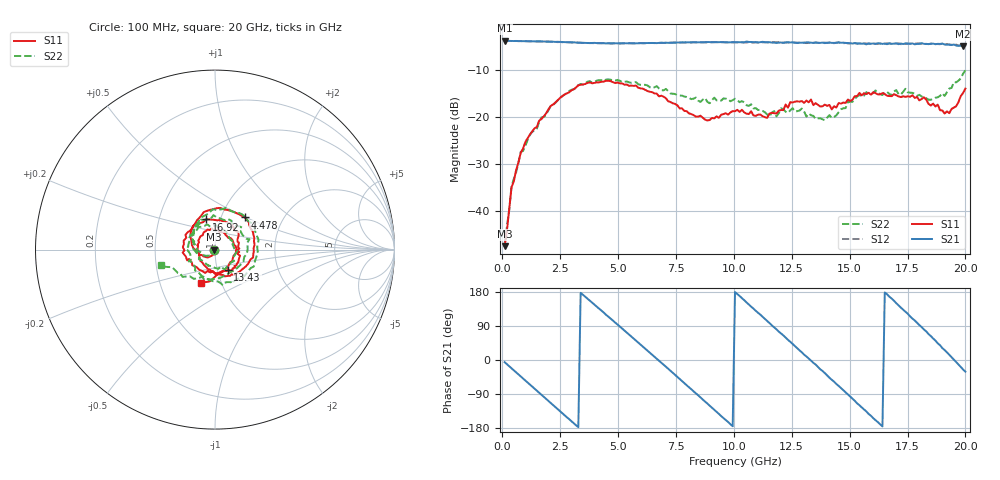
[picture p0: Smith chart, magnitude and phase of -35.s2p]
!Agilent Technologies,N5230C,MY49001569,A.09.33.09
!Agilent N5230C: A.09.33.09
!Date: Wednesday, July 29, 2015 16:57:40
!Correction: S11(Full 2 Port(1,2))
!S21(Full 2 Port(1,2))
!S12(Full 2 Port(1,2))
!S22(Full 2 Port(1,2))
!S2P File: Measurements: S11, S21, S12, S22:
# Hz S  dB  R 50
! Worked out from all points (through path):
!   201 points, 100 MHz to 20 GHz, reference 50 ohm
!   highest |S21| = -3.67 dB at 100 MHz (marker M1); lowest = -4.9 dB at 19.9 GHz (marker M2)
!   group delay of S21, straight-line fit = 153 ps
!   lowest |S11| = -47.6 dB at 100 MHz (marker M3), VSWR 1.01, Z = 49.6 - j0.0396 ohm
!   |S11| at or under -10 dB: start of sweep to end of sweep
!   |S22| runs from -47.3 to -10.0 dB; largest |S21 - S12| = 0.023
!   S11 on the Smith chart (normalised r, x): 100 MHz: 0.99, -0.00; 4.478 GHz: 1.29, +0.49; 13.43 GHz: 1.12, -0.26; 16.92 GHz: 0.86, +0.30; 20 GHz: 0.80, -0.31
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1e8  -47.59 -174.5  -3.67 -5.7  -3.65 -5.9  -47.28 -158.9
3.985e8  -34.99 -91.1  -3.77 -21.9  -3.77 -21.9  -34.74 -91.7
9.955e8  -25.33 -129.2  -3.81 -54.2  -3.80 -54.3  -26.16 -137.0
2.09e9  -17.65 168.9  -3.89 -113.4  -3.93 -113.5  -17.67 160.4
3.483e9  -13.01 95.9  -4.16 172.2  -4.18 172.2  -13.10 87.3
4.478e9  -12.27 47.4  -4.30 119.5  -4.26 119.5  -12.02 36.3
5.473e9  -13.35 1.3  -4.23 67.3  -4.26 66.8  -12.59 -9.3
6.7665e9  -15.58 -56.0  -4.18 -1.7  -4.18 -2.2  -13.90 -63.9
8.458e9  -19.93 -136.4  -4.04 -93.1  -4.03 -93.5  -16.49 -137.3
1.005e10  -18.77 116.1  -4.02 179.3  -4.08 179.3  -16.11 125.9
1.17415e10  -19.20 22.1  -4.09 86.3  -4.03 86.5  -18.74 18.8
1.2637e10  -16.73 -26.2  -4.10 36.5  -4.11 35.7  -18.82 -39.3
1.3433e10  -17.47 -57.5  -4.19 -7.4  -4.14 -7.3  -19.76 -88.8
1.4428e10  -17.98 -109.0  -4.17 -63.4  -4.10 -63.4  -19.63 -169.8
1.51245e10  -16.30 -160.2  -4.32 -102.5  -4.18 -102.4  -16.76 153.6
1.602e10  -14.70 153.7  -4.30 -153.6  -4.37 -153.0  -14.90 95.4
1.67165e10  -15.53 114.3  -4.25 167.0  -4.33 166.9  -15.08 58.6
1.69155e10  -15.14 106.2  -4.32 156.4  -4.34 154.8  -14.54 43.9
1.83085e10  -16.30 30.6  -4.41 75.5  -4.37 73.4  -16.00 -47.3
1.9005e10  -18.60 -8.6  -4.32 31.4  -4.34 30.7  -14.93 -109.4
1.99005e10  -14.87 -99.8  -4.89 -25.1  -4.84 -26.0  -10.75 -160.7
2e10  -13.94 -113.2  -4.73 -30.7  -4.97 -32.5  -10.03 -164.5
